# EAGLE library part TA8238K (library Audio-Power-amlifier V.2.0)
http://www.datasheetcatalog.org/datasheet/toshiba/1383.pdf
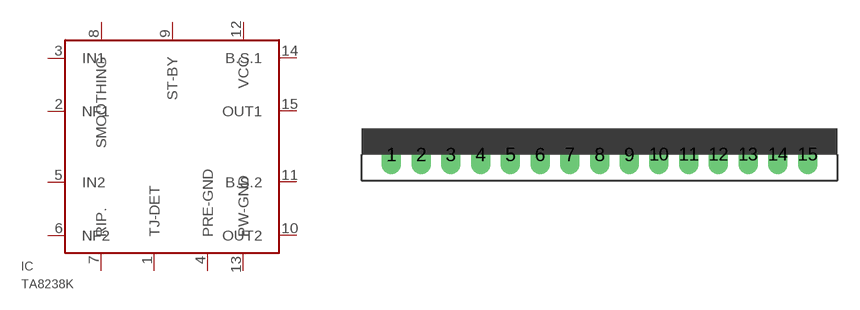
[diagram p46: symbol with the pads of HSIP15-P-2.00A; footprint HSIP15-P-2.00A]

Designator prefix IC

## TA8238K  [HSIP15-P-2.00A]
1  TJ-DET  pas
2  NF1  in
3  IN1  in
4  PRE-GND  pwr
5  IN2  in
6  NF2  in
7  RIP.  pas
8  SMOOTHING  pas
9  ST-BY  pas
10  OUT2  out
11  B.S.2  pas
12  VCC  pwr
13  PW-GND  pas
14  B.S.1  pas
15  OUT1  out

## Footprint HSIP15-P-2.00A (pad centres in mm)
drill 0.8 long: 1 -13.97,-1.27; 2 -11.97,-1.27; 3 -9.97,-1.27; 4 -7.97,-1.27; 5 -5.97,-1.27; 6 -3.97,-1.27; 7 -1.97,-1.27; 8 0.03,-1.27; 9 2.03,-1.27; 10 4.03,-1.27; 11 6.03,-1.27; 12 8.03,-1.27; 13 10.03,-1.27; 14 12.03,-1.27; 15 14.03,-1.27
